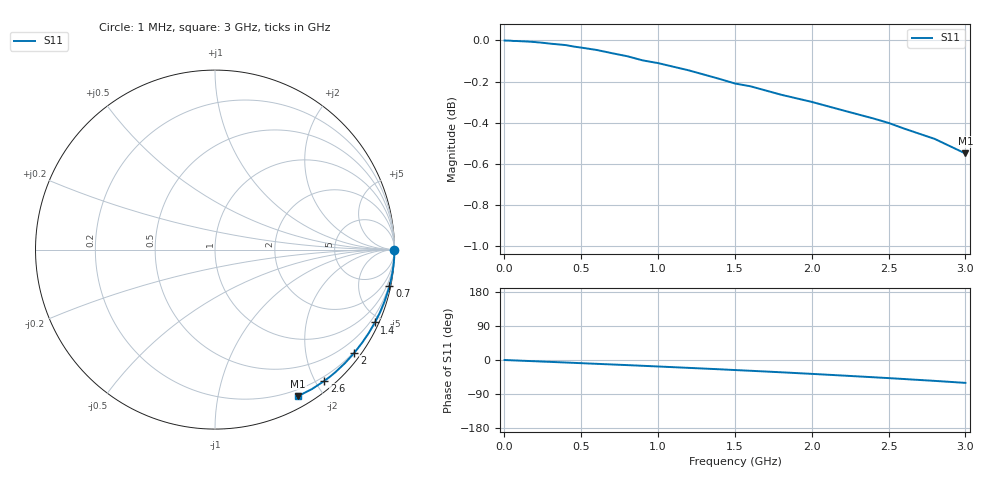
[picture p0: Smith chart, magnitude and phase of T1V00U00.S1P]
! SIEMENS Small Signal Semiconductors
! BAT68-04
! Si Schottky Diode (2 diodes in series, pin 3 open) in SOT23
! VR = 0 V
! S-Parameters:  August  1994
# GHz  S  MA  R  50
!  f  S11
! GHz  MAG  ANG
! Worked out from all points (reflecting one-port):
!   33 points, 1 MHz to 3 GHz, reference 50 ohm
!   lowest |S11| = -0.5 dB at 3 GHz (marker M1), VSWR 31.63, Z = 6.23 - j85.6 ohm
!   phase of S11 starts at 0 deg and turns -60 deg over the sweep
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0.001  1 0.0
0.003  1 0.0
0.01  0.9999 -0.2
0.05  0.9998 -0.8
0.08  0.9997 -1.3
0.1  0.9996 -1.7
0.2  0.9991 -3.3
0.25  0.9987 -4.2
0.35  0.9978 -5.8
0.4  0.9974 -6.7
0.45  0.9966 -7.5
0.5  0.996 -8.4
0.6  0.9947 -10.1
0.7  0.9929 -11.8
0.8  0.9912 -13.5
1  0.9874 -17.1
1.2  0.9834 -20.8
1.4  0.9787 -24.5
1.5  0.9762 -26.5
1.6  0.9747 -28.4
1.8  0.9701 -32.4
2  0.9662 -36.6
2.2  0.9617 -41.0
2.4  0.9573 -45.5
2.5  0.9549 -47.8
2.6  0.9519 -50.2
2.8  0.9464 -55.1
3  0.9387 -60.4
